|   TEXAS INSTRUMENTS INCORPORATION
|   Package IBIS MODEL 144 PGE Package
[IBIS Ver]   2.1
[File Name]   sprm255.ibs
[File Rev]   1.0
[Date]   April 03, 2001
[Source]   IBIS Model Generated from PACED 4.40B
[Notes]
[Disclaimer]   Please be aware that in the absence of a written agreement
|   Texas Instruments(TI) assumes no liability for:
|   (1) The accuracy of the IBIS models provided to your company
|   (2) The proper functioning of these Models in your design
|   or for any resulting applications;or
|   (3)Infringement of patents,copyrights or intellectual
|   property rights resulting from your use of these models.
|   TI provides IBIS Models as a service to our customers and
|   therefore reserves the right to limit distribution of the
|   Models.
[Copyright]   Property of Texas Instruments Incorporated.
|   Unauthorised reproduction and/or distribution is strictly
|   prohibited.
|   This product is protected under copyright law and trade
|   secret law as an unpublished work.
|   Created 1999,(C) Copyright 1999-2001,
|   Texas Instruments Incorporated., All Rights Reserved.
|   These commodities are under the U.S.
|   Government distribution license control.As such,they are not
|   to be re-exported without the prior approval of the U.S.
|   Department of Commerce.
[component]   F741724
[Manufacturer]   Texas Instruments Inc.
[Package]
| Variable   Typ   Min   Max
R_pkg   0.152   0.1207   0.1617
L_pkg   7.844e-09   7.096e-09   9.059e-09
C_pkg   1.205e-12   1.076e-12   1.386e-12
[Pin]   signal_name  model_name   R_pin   L_pin   C_pin
1   GND   GND   0.1583   9.041e-09   1.136e-12
2   PA22   OUK831/UPS239  0.157   8.742e-09   1.384e-12
3   GND   GND   0.1567   8.585e-09   1.359e-12
4   POWER   POWER   0.1556   8.418e-09   1.335e-12
5   A10   OUK831/UPS239  0.1548   8.278e-09   1.27e-12
6   HD7   OUK831/UPS239  0.1541   8.14e-09   1.243e-12
7   A11   OUK831/UPS239  0.1535   7.997e-09   1.263e-12
8   A12   OUK831/UPS239  0.1529   7.871e-09   1.247e-12
9   A13   OUK831/UPS239  0.1524   7.76e-09   1.206e-12
10   A14   OUK831/UPS239  0.1531   7.712e-09   1.149e-12
11   A15   OUK831/UPS239  0.1521   7.58e-09   1.154e-12
12   POWER   POWER   0.1218   7.353e-09   1.176e-12
13   HAS_   IDG091_PS1001  0.1512   7.383e-09   1.143e-12
14   GND   GND   0.1512   7.332e-09   1.119e-12
15   GND   GND   0.151   7.273e-09   1.094e-12
16   POWER   POWER   0.1207   7.096e-09   1.098e-12
17   HCS_   IDG091_PS1001  0.1508   7.237e-09   1.085e-12
18   HRW   IDG041_PS1001  0.1507   7.257e-09   1.276e-12
19   READY   IDG041   0.1497   7.25e-09   1.273e-12
20   PS_   OUK831   0.15   7.234e-09   1.077e-12
21   DS_   OUK831   0.1502   7.216e-09   1.076e-12
22   IS_   OUK831   0.1507   7.272e-09   1.087e-12
23   RW_   OUK831   0.1511   7.329e-09   1.115e-12
24   MSTRB_   OUK831   0.1513   7.383e-09   1.137e-12
25   IOSTRB_   OUK831   0.1521   7.479e-09   1.145e-12
26   MSC_   OUK831   0.1519   7.558e-09   1.135e-12
27   XF   OUK831   0.153   7.681e-09   1.155e-12
28   HOLDA_   OUK831   0.1533   7.758e-09   1.216e-12
29   IAQ_   OUK831   0.1541   7.872e-09   1.245e-12
30   HOLD_   IDG041   0.1549   7.999e-09   1.26e-12
31   BIO_   IDG091   0.1559   8.143e-09   1.242e-12
32   MPNMC_   IDG041   0.1573   8.302e-09   1.268e-12
33   POWER   POWER   0.1583   8.441e-09   1.334e-12
34   GND   GND   0.1595   8.606e-09   1.36e-12
35   BDR1   IDG041   0.1602   8.765e-09   1.386e-12
36   BFSR1   OUK831/IDG041  0.1617   9.059e-09   1.137e-12
37   GND   GND   0.1583   9.041e-09   1.136e-12
38   BCLKR1   OUK831/IDG091  0.157   8.742e-09   1.384e-12
39   HCNTL0   IDG041_PS1001  0.1567   8.585e-09   1.359e-12
40   GND   GND   0.1556   8.418e-09   1.335e-12
41   BCLKR0   OUK831/IDG091  0.1548   8.278e-09   1.27e-12
42   BCLKR2   OUK831/IDG091  0.1541   8.14e-09   1.243e-12
43   BFSR0   OUK831/IDG041  0.1535   7.997e-09   1.263e-12
44   BFSR2   OUK831/IDG041  0.1529   7.871e-09   1.247e-12
45   BDR0   IDG041   0.1524   7.76e-09   1.206e-12
46   HCNTL1   IDG041_PS1001  0.1531   7.712e-09   1.149e-12
47   BDR2   IDG041   0.1521   7.583e-09   1.152e-12
48   BCLKX0   OUK831/IDG091  0.1517   7.479e-09   1.159e-12
49   BCLKX2   OUK831/IDG091  0.1512   7.386e-09   1.14e-12
50   GND   GND   0.1512   7.333e-09   1.119e-12
51   HINT   OUK831   0.151   7.276e-09   1.091e-12
52   POWER   POWER   0.1508   7.222e-09   1.081e-12
53   BFSX0   OUK831/IDG041  0.1508   7.24e-09   1.083e-12
54   BFSX2   OUK831/IDG041  0.1507   7.258e-09   1.276e-12
55   HRDY   OUK831   0.1497   7.25e-09   1.273e-12
56   POWER   POWER   0.15   7.234e-09   1.077e-12
57   GND   GND   0.1502   7.216e-09   1.076e-12
58   HD0   OUK831/UPS239  0.1507   7.272e-09   1.087e-12
59   BDX0   OUK831   0.1511   7.329e-09   1.115e-12
60   BDX2   OUK831   0.1513   7.383e-09   1.137e-12
61   IACK_   OUK831   0.1521   7.479e-09   1.145e-12
62   HBIL   IDG041_PS1001  0.1519   7.558e-09   1.135e-12
63   NMI_   IDG091   0.153   7.681e-09   1.155e-12
64   INT0_   IDG091   0.1533   7.758e-09   1.216e-12
65   INT1_   IDG091   0.1541   7.872e-09   1.245e-12
66   INT2_   IDG091   0.1549   7.999e-09   1.26e-12
67   INT3_   IDG091   0.1559   8.143e-09   1.242e-12
68   POWER   POWER   0.1573   8.302e-09   1.268e-12
69   HD1   OUK831/UPS239  0.1583   8.441e-09   1.334e-12
70   GND   GND   0.1595   8.606e-09   1.36e-12
71   BCLKX1   OUK831/IDG091  0.1602   8.765e-09   1.386e-12
72   GND   GND   0.1617   9.059e-09   1.137e-12
73   BFSX1   OUK831/IDG041  0.1583   9.041e-09   1.136e-12
74   BDX1   OUK831   0.157   8.742e-09   1.384e-12
75   POWER   POWER   0.1567   8.585e-09   1.359e-12
76   GND   GND   0.1556   8.418e-09   1.335e-12
77   CLKMD1   IDG091   0.1548   8.278e-09   1.27e-12
78   CLKMD2   IDG091   0.1541   8.14e-09   1.243e-12
79   CLKMD3   IDG091   0.1535   7.997e-09   1.263e-12
80   HPI16   IDG041_PE1001  0.1529   7.871e-09   1.247e-12
81   HD2   OUK831/UPS239  0.1524   7.76e-09   1.206e-12
82   TOUT   OUK831   0.1531   7.712e-09   1.149e-12
83   EMU0   OUK831/IDG041  0.1521   7.583e-09   1.152e-12
84   EMU1   OUK831/IDG041  0.1517   7.479e-09   1.159e-12
85   TDO   OUK831   0.1512   7.386e-09   1.14e-12
86   TDI   IDG041_PS1001  0.1512   7.333e-09   1.119e-12
87   TRST_   IDG041_PE1001  0.151   7.276e-09   1.091e-12
88   TCK   IDG091_PS1001  0.1508   7.222e-09   1.081e-12
89   TMS   IDG041_PS1001  0.1508   7.24e-09   1.083e-12
90   GND   GND   0.1507   7.258e-09   1.281e-12
91   POWER   POWER   0.1198   7.122e-09   1.29e-12
92   HPIENA   IDG041_PE1001  0.15   7.231e-09   1.08e-12
93   GND   GND   0.1502   7.215e-09   1.076e-12
94   CLKOUT   OUKB31   0.1507   7.271e-09   1.087e-12
95   HD3   OUK831/UPS239  0.1511   7.329e-09   1.115e-12
96   X1   NC   0.1513   7.383e-09   1.137e-12
97   X2CLKIN   UIS434   0.1521   7.479e-09   1.145e-12
98   RS_   IDG041   0.1519   7.558e-09   1.135e-12
99   D0   OUK831/UPS239  0.153   7.681e-09   1.155e-12
100   D1   OUK831/UPS239  0.1533   7.758e-09   1.216e-12
101   D2   OUK831/UPS239  0.1541   7.872e-09   1.245e-12
102   D3   OUK831/UPS239  0.1549   7.999e-09   1.26e-12
103   D4   OUK831/UPS239  0.1559   8.143e-09   1.242e-12
104   D5   OUK831/UPS239  0.1573   8.302e-09   1.268e-12
105   PA16   OUK831/UPS239  0.1583   8.441e-09   1.334e-12
106   GND   GND   0.1595   8.606e-09   1.36e-12
107   PA17   OUK831   0.1602   8.765e-09   1.386e-12
108   PA18   OUK831   0.1617   9.059e-09   1.137e-12
109   PA19   OUK831   0.1583   9.041e-09   1.136e-12
110   PA20   OUK831   0.157   8.742e-09   1.384e-12
111   GND   GND   0.1567   8.585e-09   1.359e-12
112   POWER   POWER   0.1556   8.418e-09   1.335e-12
113   D6   OUK831/UPS239  0.1548   8.278e-09   1.27e-12
114   D7   OUK831/UPS239  0.1541   8.14e-09   1.243e-12
115   D8   OUK831/UPS239  0.1535   7.997e-09   1.263e-12
116   D9   OUK831/UPS239  0.1529   7.871e-09   1.247e-12
117   D10   OUK831/UPS239  0.1524   7.76e-09   1.206e-12
118   D11   OUK831/UPS239  0.1531   7.712e-09   1.149e-12
119   D12   OUK831/UPS239  0.1521   7.583e-09   1.152e-12
120   HD4   OUK831/UPS239  0.1517   7.479e-09   1.159e-12
121   D13   OUK831/UPS239  0.1512   7.386e-09   1.141e-12
122   D14   OUK831/UPS239  0.1512   7.333e-09   1.119e-12
123   D15   OUK831/UPS239  0.151   7.275e-09   1.092e-12
124   HD5   OUK831/UPS239  0.1507   7.219e-09   1.083e-12
125   POWER   POWER   0.1208   7.114e-09   1.1e-12
126   GND   GND   0.1507   7.255e-09   1.278e-12
127   HDS1   IDG091_PS1001  0.1497   7.25e-09   1.273e-12
128   GND   GND   0.15   7.234e-09   1.077e-12
129   HDS2   IDG091_PS1001  0.1502   7.216e-09   1.076e-12
130   POWER   POWER   0.1507   7.272e-09   1.087e-12
131   A0   OUK831/UPS239  0.1511   7.329e-09   1.115e-12
132   A1   OUK831/UPS239  0.1513   7.383e-09   1.137e-12
133   A2   OUK831/UPS239  0.1521   7.479e-09   1.145e-12
134   A3   OUK831/UPS239  0.1519   7.558e-09   1.135e-12
135   HD6   OUK831/UPS239  0.153   7.681e-09   1.155e-12
136   A4   OUK831/UPS239  0.1533   7.758e-09   1.216e-12
137   A5   OUK831/UPS239  0.1541   7.871e-09   1.245e-12
138   A6   OUK831/UPS239  0.1549   7.998e-09   1.26e-12
139   A7   OUK831/UPS239  0.1559   8.143e-09   1.242e-12
140   A8   OUK831/UPS239  0.1573   8.301e-09   1.268e-12
141   A9   OUK831/UPS239  0.1583   8.437e-09   1.337e-12
142   POWER   POWER   0.1287   8.462e-09   1.381e-12
143   PA21   OUK831   0.1602   8.76e-09   1.389e-12
144   GND   GND   0.1617   9.058e-09   1.137e-12
[Component]   UIS434
[Manufacturer]   Texas Instruments
[Package]
|   typ   min   max
R_pkg   0   0   0
L_pkg   0   0   0
C_pkg   0   0   0
[Pin]   signal_name   model_name   R_pin   L_pin   C_pin
   1   XI   UIS434   0   0   0
[Component]   IDG091
[Manufacturer]   Texas Instruments
[Package]
|   typ   min   max
R_pkg   0   0   0
L_pkg   0   0   0
C_pkg   0   0   0
[Pin]   signal_name   model_name   R_pin   L_pin   C_pin
   1   A   IDG091   0   0   0
[Component]   IDG041_PE1001
[Manufacturer]   Texas Instruments
[Package]
|   typ   min   max
R_pkg   0   0   0
L_pkg   0   0   0
C_pkg   0   0   0
[Pin]   signal_name   model_name   R_pin   L_pin   C_pin
   1   A   IDG041_PE1001   0   0   0
[Component]   IDG041
[Manufacturer]   Texas Instruments
[Package]
|   typ   min   max
R_pkg   0   0   0
L_pkg   0   0   0
C_pkg   0   0   0
[Pin]   signal_name   model_name   R_pin   L_pin   C_pin
   1   A   IDG041   0   0   0
[Component]   IDG041_PS1001
[Manufacturer]   Texas Instruments
[Package]
|   typ   min   max
R_pkg   0   0   0
L_pkg   0   0   0
C_pkg   0   0   0
[Pin]   signal_name   model_name   R_pin   L_pin   C_pin
   1   A   IDG041_PS1001   0   0   0
[Component]   IDG091_PS1001
[Manufacturer]   Texas Instruments
[Package]
|   typ   min   max
R_pkg   0   0   0
L_pkg   0   0   0
C_pkg   0   0   0
[Pin]   signal_name   model_name   R_pin   L_pin   C_pin
   1   A   IDG091_PS1001   0   0   0
[Component]   OUK831
[Manufacturer]   Texas Instruments
[Package]
|   typ   min   max
R_pkg   0   0   0
L_pkg   0   0   0
C_pkg   0   0   0
[Pin]   signal_name   model_name   R_pin   L_pin   C_pin
   1   Y   OUK831   0   0   0
[Component]   OUKB31
[Manufacturer]   Texas Instruments
[Package]
|   typ   min   max
R_pkg   0   0   0
L_pkg   0   0   0
C_pkg   0   0   0
[Pin]   signal_name   model_name   R_pin   L_pin   C_pin
   1   Y   OUKB31   0   0   0
[Component]   UPS239
[Manufacturer]   Texas Instruments
[Package]
|   typ   min   max
R_pkg   0   0   0
L_pkg   0   0   0
C_pkg   0   0   0
[Pin]   signal_name   model_name   R_pin   L_pin   C_pin
   1   A   UPS239   0   0   0
| Models and submodels in the file (9): UIS434 (Input), IDG091 (Input), IDG041_PE1001 (Input), IDG041 (Input), IDG041_PS1001 (Input), IDG091_PS1001 (Input), OUK831 (3-state), OUKB31 (3-state), UPS239 (Input)
